{attribute 'call_after_init'}
FUNCTION_BLOCK FB_DS_IED_LD1_LLN0_DS8 EXTENDS FB_AcsiCommonDataSetClass
VAR
END_VAR

METHOD OnInit : BOOL
VAR
END_VAR
IF NOT DeleteAllMembers() THEN RETURN; END_IF
IF NOT AddMember(ipData:=fbIED.IEDLD1.LPHD1.PhyNam, eFc:=E_AcsiFc.DC) THEN RETURN; END_IF
IF NOT AddMember(ipData:=fbIED.IEDLD1.LLN0.NamPlt, eFc:=E_AcsiFc.DC) THEN RETURN; END_IF
IF NOT AddMember(ipData:=fbIED.IEDLD1.MMXU1.NamPlt, eFc:=E_AcsiFc.DC) THEN RETURN; END_IF
IF NOT AddMember(ipData:=fbIED.IEDLD1.XCBR1.NamPlt, eFc:=E_AcsiFc.DC) THEN RETURN; END_IF
IF NOT AddMember(ipData:=fbIED.IEDLD1.CSWI1.NamPlt, eFc:=E_AcsiFc.DC) THEN RETURN; END_IF
IF NOT AddMember(ipData:=fbIED.IEDLD1.LEDGGIO1.NamPlt, eFc:=E_AcsiFc.DC) THEN RETURN; END_IF
IF NOT AddMember(ipData:=fbIED.IEDLD1.LEDGGIO2.NamPlt, eFc:=E_AcsiFc.DC) THEN RETURN; END_IF
IF NOT AddMember(ipData:=fbIED.IEDLD1.LEDGGIO3.NamPlt, eFc:=E_AcsiFc.DC) THEN RETURN; END_IF
IF NOT AddMember(ipData:=fbIED.IEDLD1.LEDGGIO4.NamPlt, eFc:=E_AcsiFc.DC) THEN RETURN; END_IF
IF NOT AddMember(ipData:=fbIED.IEDLD1.LEDGGIO5.NamPlt, eFc:=E_AcsiFc.DC) THEN RETURN; END_IF
IF NOT AddMember(ipData:=fbIED.IEDLD1.LEDGGIO6.NamPlt, eFc:=E_AcsiFc.DC) THEN RETURN; END_IF
IF NOT AddMember(ipData:=fbIED.IEDLD1.LEDGGIO7.NamPlt, eFc:=E_AcsiFc.DC) THEN RETURN; END_IF
IF NOT AddMember(ipData:=fbIED.IEDLD1.LEDGGIO8.NamPlt, eFc:=E_AcsiFc.DC) THEN RETURN; END_IF
IF NOT AddMember(ipData:=fbIED.IEDLD1.ATCC1.NamPlt, eFc:=E_AcsiFc.DC) THEN RETURN; END_IF
OnInit:= TRUE;
END_METHOD

END_FUNCTION_BLOCK
